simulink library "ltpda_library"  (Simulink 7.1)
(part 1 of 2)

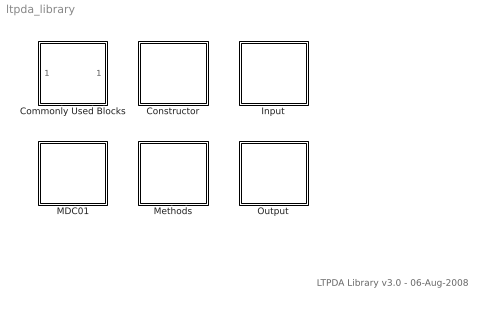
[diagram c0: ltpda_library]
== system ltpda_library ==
  note: LTPDA Library v3.0 - 06-Aug-2008
  Commonly Used Blocks : Subsystem
  Constructor : Subsystem  Tag=subsystem  AncestorBlock=libraryBase/SubSystName
  Input : Subsystem
  MDC01 : Subsystem  Tag=subsystem  AncestorBlock=libraryBase/SubSystName
  Methods : Subsystem  Tag=subsystem  AncestorBlock=libraryBase/SubSystName
  Output : Subsystem

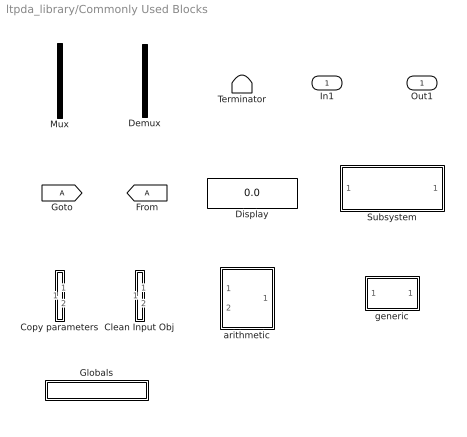
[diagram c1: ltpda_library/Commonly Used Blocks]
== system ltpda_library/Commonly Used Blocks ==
  In1 : Inport  OutDataType=sfix(16)  OutScaling=2^0
  Clean Input Obj : Subsystem
  Copy parameters : Subsystem
  Demux : Demux  Tag=demux  Outputs=2
  Display : Display
  Globals : Subsystem  Tag=globals
  Mux : Mux  Tag=mux  Inputs=2
  Subsystem : Subsystem
  Terminator : Terminator
  arithmetic : Subsystem  Tag=arithmetic
  generic : Subsystem  Tag=function
  Out1 : Outport  OutDataType=sfix(16)  OutScaling=2^0

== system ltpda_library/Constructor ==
  ltpda_getAOsInTimeSpan : Subsystem  Tag=function  AncestorBlock=libraryBase/function

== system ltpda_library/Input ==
  Object from list : Subsystem  Tag=input

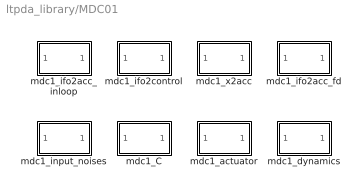
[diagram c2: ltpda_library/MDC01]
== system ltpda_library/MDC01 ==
  mdc1_C : Subsystem  Tag=function  AncestorBlock=libraryBase/function
  mdc1_actuator : Subsystem  Tag=function  AncestorBlock=libraryBase/function
  mdc1_dynamics : Subsystem  Tag=function  AncestorBlock=libraryBase/function
  mdc1_ifo2acc_fd : Subsystem  Tag=function  AncestorBlock=libraryBase/function
  mdc1_ifo2acc_inloop : Subsystem  Tag=function  AncestorBlock=libraryBase/function
  mdc1_ifo2control : Subsystem  Tag=function  AncestorBlock=libraryBase/function
  mdc1_input_noises : Subsystem  Tag=function  AncestorBlock=libraryBase/function
  mdc1_x2acc : Subsystem  Tag=function  AncestorBlock=libraryBase/function

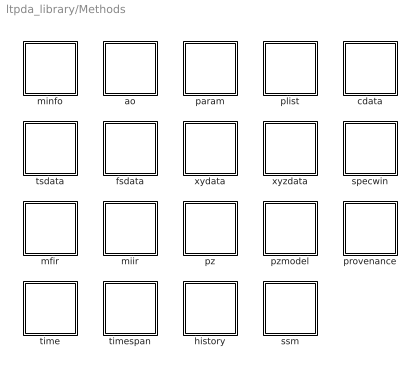
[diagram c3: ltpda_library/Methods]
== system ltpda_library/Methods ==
  ao : Subsystem  Tag=subsystem  AncestorBlock=libraryBase/SubSystName
  cdata : Subsystem  Tag=subsystem  AncestorBlock=libraryBase/SubSystName
  fsdata : Subsystem  Tag=subsystem  AncestorBlock=libraryBase/SubSystName
  history : Subsystem  Tag=subsystem  AncestorBlock=libraryBase/SubSystName
  mfir : Subsystem  Tag=subsystem  AncestorBlock=libraryBase/SubSystName
  miir : Subsystem  Tag=subsystem  AncestorBlock=libraryBase/SubSystName
  minfo : Subsystem  Tag=subsystem  AncestorBlock=libraryBase/SubSystName
  param : Subsystem  Tag=subsystem  AncestorBlock=libraryBase/SubSystName
  plist : Subsystem  Tag=subsystem  AncestorBlock=libraryBase/SubSystName
  provenance : Subsystem  Tag=subsystem  AncestorBlock=libraryBase/SubSystName
  pz : Subsystem  Tag=subsystem  AncestorBlock=libraryBase/SubSystName
  pzmodel : Subsystem  Tag=subsystem  AncestorBlock=libraryBase/SubSystName
  specwin : Subsystem  Tag=subsystem  AncestorBlock=libraryBase/SubSystName
  ssm : Subsystem  Tag=subsystem  AncestorBlock=libraryBase/SubSystName
  time : Subsystem  Tag=subsystem  AncestorBlock=libraryBase/SubSystName
  timespan : Subsystem  Tag=subsystem  AncestorBlock=libraryBase/SubSystName
  tsdata : Subsystem  Tag=subsystem  AncestorBlock=libraryBase/SubSystName
  xydata : Subsystem  Tag=subsystem  AncestorBlock=libraryBase/SubSystName
  xyzdata : Subsystem  Tag=subsystem  AncestorBlock=libraryBase/SubSystName

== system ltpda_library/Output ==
  Send to output : Subsystem
  iplot : Subsystem  Tag=method ao
  plot : Subsystem  Tag=method ao
  save : Subsystem  Tag=method ao

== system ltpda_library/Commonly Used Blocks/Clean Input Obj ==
  In1 : Inport  OutDataType=sfix(16)  OutScaling=2^0
  In2 : Inport  Port=2  OutDataType=sfix(16)  OutScaling=2^0
  cleaninput : M-S-Function  FunctionName=g_cleaninput
  Out1 : Outport  OutDataType=sfix(16)  OutScaling=2^0
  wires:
  In2/1 -> cleaninput/2
  In1/1 -> cleaninput/1
  cleaninput/1 -> Out1/1

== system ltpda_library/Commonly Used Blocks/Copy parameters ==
  In1 : Inport  OutDataType=sfix(16)  OutScaling=2^0
  In2 : Inport  Port=2  OutDataType=sfix(16)  OutScaling=2^0
  copyparam : M-S-Function  FunctionName=g_copyparams
  Out1 : Outport  OutDataType=sfix(16)  OutScaling=2^0
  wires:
  copyparam/1 -> Out1/1
  In1/1 -> copyparam/1
  In2/1 -> copyparam/2

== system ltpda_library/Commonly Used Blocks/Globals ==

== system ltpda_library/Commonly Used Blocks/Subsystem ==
  In1 : Inport  OutDataType=sfix(16)  OutScaling=2^0
  Out1 : Outport  OutDataType=sfix(16)  OutScaling=2^0

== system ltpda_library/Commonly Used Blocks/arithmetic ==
  alpha : Inport  Tag=1  OutDataType=sfix(16)  OutScaling=2^0
  beta : Inport  Tag=2  Port=2  OutDataType=sfix(16)  OutScaling=2^0
  Mux : Mux  Tag=mux  Inputs=2
  arithmetic_func : M-S-Function  Tag=arithmetic  FunctionName=ltpdasim
  Out1 : Outport  OutDataType=sfix(16)  OutScaling=2^0
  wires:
  arithmetic_func/1 -> Out1/1
  Mux/1 -> arithmetic_func/1
  alpha/1 -> Mux/1
  beta/1 -> Mux/2

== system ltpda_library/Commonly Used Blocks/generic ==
  In1 : Inport  OutDataType=sfix(16)  OutScaling=2^0
  generic : M-S-Function  Tag=generic  FunctionName=ltpdasim
  Out1 : Outport  OutDataType=sfix(16)  OutScaling=2^0
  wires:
  generic/1 -> Out1/1
  In1/1 -> generic/1

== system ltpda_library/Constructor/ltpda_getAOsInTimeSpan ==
  In1 : Inport  OutDataType=sfix(16)  OutScaling=2^0
  ltpda_getAOsInTimeSpan : M-S-Function  Tag=ltpda_getAOsInTimeSpan  FunctionName=ltpdasim
  Out1 : Outport  OutDataType=sfix(16)  OutScaling=2^0
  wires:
  In1/1 -> ltpda_getAOsInTimeSpan/1
  ltpda_getAOsInTimeSpan/1 -> Out1/1

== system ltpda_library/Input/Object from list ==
  Input : Constant  Value=0  OutDataType=sfix(16)  OutScaling=2^0
  Input AO : Outport  OutDataType=sfix(16)  OutScaling=2^0
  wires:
  Input/1 -> Input AO/1

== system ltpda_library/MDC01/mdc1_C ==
  In1 : Inport  OutDataType=sfix(16)  OutScaling=2^0
  ltpda_mdc1_C : M-S-Function  Tag=ltpda_mdc1_C  FunctionName=ltpdasim
  Out1 : Outport  OutDataType=sfix(16)  OutScaling=2^0
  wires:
  In1/1 -> ltpda_mdc1_C/1
  ltpda_mdc1_C/1 -> Out1/1

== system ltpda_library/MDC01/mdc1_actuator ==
  In1 : Inport  OutDataType=sfix(16)  OutScaling=2^0
  ltpda_mdc1_actuator : M-S-Function  Tag=ltpda_mdc1_actuator  FunctionName=ltpdasim
  Out1 : Outport  OutDataType=sfix(16)  OutScaling=2^0
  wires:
  In1/1 -> ltpda_mdc1_actuator/1
  ltpda_mdc1_actuator/1 -> Out1/1

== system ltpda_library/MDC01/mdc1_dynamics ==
  In1 : Inport  OutDataType=sfix(16)  OutScaling=2^0
  ltpda_mdc1_dynamics : M-S-Function  Tag=ltpda_mdc1_dynamics  FunctionName=ltpdasim
  Out1 : Outport  OutDataType=sfix(16)  OutScaling=2^0
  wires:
  In1/1 -> ltpda_mdc1_dynamics/1
  ltpda_mdc1_dynamics/1 -> Out1/1

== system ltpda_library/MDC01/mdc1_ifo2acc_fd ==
  In1 : Inport  OutDataType=sfix(16)  OutScaling=2^0
  ltpda_mdc1_ifo2acc_fd : M-S-Function  Tag=ltpda_mdc1_ifo2acc_fd  FunctionName=ltpdasim
  Out1 : Outport  OutDataType=sfix(16)  OutScaling=2^0
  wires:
  In1/1 -> ltpda_mdc1_ifo2acc_fd/1
  ltpda_mdc1_ifo2acc_fd/1 -> Out1/1

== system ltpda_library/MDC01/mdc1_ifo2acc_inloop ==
  In1 : Inport  OutDataType=sfix(16)  OutScaling=2^0
  ltpda_mdc1_ifo2acc_inloop : M-S-Function  Tag=ltpda_mdc1_ifo2acc_inloop  FunctionName=ltpdasim
  Out1 : Outport  OutDataType=sfix(16)  OutScaling=2^0
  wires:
  In1/1 -> ltpda_mdc1_ifo2acc_inloop/1
  ltpda_mdc1_ifo2acc_inloop/1 -> Out1/1

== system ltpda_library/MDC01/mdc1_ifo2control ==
  In1 : Inport  OutDataType=sfix(16)  OutScaling=2^0
  ltpda_mdc1_ifo2control : M-S-Function  Tag=ltpda_mdc1_ifo2control  FunctionName=ltpdasim
  Out1 : Outport  OutDataType=sfix(16)  OutScaling=2^0
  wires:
  In1/1 -> ltpda_mdc1_ifo2control/1
  ltpda_mdc1_ifo2control/1 -> Out1/1

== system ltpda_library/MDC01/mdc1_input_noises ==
  In1 : Inport  OutDataType=sfix(16)  OutScaling=2^0
  ltpda_mdc1_input_noises : M-S-Function  Tag=ltpda_mdc1_input_noises  FunctionName=ltpdasim
  Out1 : Outport  OutDataType=sfix(16)  OutScaling=2^0
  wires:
  In1/1 -> ltpda_mdc1_input_noises/1
  ltpda_mdc1_input_noises/1 -> Out1/1

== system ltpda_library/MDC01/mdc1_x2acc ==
  In1 : Inport  OutDataType=sfix(16)  OutScaling=2^0
  ltpda_mdc1_x2acc : M-S-Function  Tag=ltpda_mdc1_x2acc  FunctionName=ltpdasim
  Out1 : Outport  OutDataType=sfix(16)  OutScaling=2^0
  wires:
  In1/1 -> ltpda_mdc1_x2acc/1
  ltpda_mdc1_x2acc/1 -> Out1/1

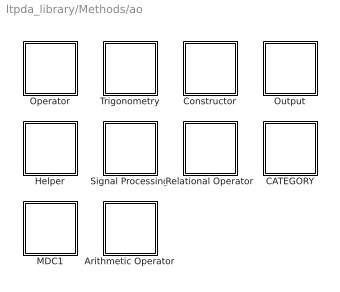
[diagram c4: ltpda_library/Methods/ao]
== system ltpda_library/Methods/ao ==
  Arithmetic Operator : Subsystem  Tag=subsystem  AncestorBlock=libraryBase/SubSystName
  CATEGORY : Subsystem  Tag=subsystem  AncestorBlock=libraryBase/SubSystName
  Constructor : Subsystem  Tag=subsystem  AncestorBlock=libraryBase/SubSystName
  Helper : Subsystem  Tag=subsystem  AncestorBlock=libraryBase/SubSystName
  MDC1 : Subsystem  Tag=subsystem  AncestorBlock=libraryBase/SubSystName
  Operator : Subsystem  Tag=subsystem  AncestorBlock=libraryBase/SubSystName
  Output : Subsystem  Tag=subsystem  AncestorBlock=libraryBase/SubSystName
  Relational Operator : Subsystem  Tag=subsystem  AncestorBlock=libraryBase/SubSystName
  Signal Processing : Subsystem  Tag=subsystem  AncestorBlock=libraryBase/SubSystName
  Trigonometry : Subsystem  Tag=subsystem  AncestorBlock=libraryBase/SubSystName

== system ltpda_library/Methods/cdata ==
  Constructor : Subsystem  Tag=subsystem  AncestorBlock=libraryBase/SubSystName
  Output : Subsystem  Tag=subsystem  AncestorBlock=libraryBase/SubSystName

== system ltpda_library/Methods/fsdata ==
  Constructor : Subsystem  Tag=subsystem  AncestorBlock=libraryBase/SubSystName
  Output : Subsystem  Tag=subsystem  AncestorBlock=libraryBase/SubSystName

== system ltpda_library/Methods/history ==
  Constructor : Subsystem  Tag=subsystem  AncestorBlock=libraryBase/SubSystName
  Output : Subsystem  Tag=subsystem  AncestorBlock=libraryBase/SubSystName

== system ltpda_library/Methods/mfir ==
  Constructor : Subsystem  Tag=subsystem  AncestorBlock=libraryBase/SubSystName
  Helper : Subsystem  Tag=subsystem  AncestorBlock=libraryBase/SubSystName
  Output : Subsystem  Tag=subsystem  AncestorBlock=libraryBase/SubSystName
  Signal Processing : Subsystem  Tag=subsystem  AncestorBlock=libraryBase/SubSystName

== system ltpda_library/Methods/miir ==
  Constructor : Subsystem  Tag=subsystem  AncestorBlock=libraryBase/SubSystName
  Helper : Subsystem  Tag=subsystem  AncestorBlock=libraryBase/SubSystName
  Output : Subsystem  Tag=subsystem  AncestorBlock=libraryBase/SubSystName
  Signal Processing : Subsystem  Tag=subsystem  AncestorBlock=libraryBase/SubSystName

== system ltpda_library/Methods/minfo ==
  Constructor : Subsystem  Tag=subsystem  AncestorBlock=libraryBase/SubSystName
  Output : Subsystem  Tag=subsystem  AncestorBlock=libraryBase/SubSystName

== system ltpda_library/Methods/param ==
  Constructor : Subsystem  Tag=subsystem  AncestorBlock=libraryBase/SubSystName
  Helper : Subsystem  Tag=subsystem  AncestorBlock=libraryBase/SubSystName
  Output : Subsystem  Tag=subsystem  AncestorBlock=libraryBase/SubSystName

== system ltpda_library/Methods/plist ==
  Constructor : Subsystem  Tag=subsystem  AncestorBlock=libraryBase/SubSystName
  Helper : Subsystem  Tag=subsystem  AncestorBlock=libraryBase/SubSystName
  Output : Subsystem  Tag=subsystem  AncestorBlock=libraryBase/SubSystName
  Signal Processing : Subsystem  Tag=subsystem  AncestorBlock=libraryBase/SubSystName

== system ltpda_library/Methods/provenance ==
  Constructor : Subsystem  Tag=subsystem  AncestorBlock=libraryBase/SubSystName
  Output : Subsystem  Tag=subsystem  AncestorBlock=libraryBase/SubSystName

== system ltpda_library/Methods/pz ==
  Constructor : Subsystem  Tag=subsystem  AncestorBlock=libraryBase/SubSystName
  Output : Subsystem  Tag=subsystem  AncestorBlock=libraryBase/SubSystName
  Signal Processing : Subsystem  Tag=subsystem  AncestorBlock=libraryBase/SubSystName

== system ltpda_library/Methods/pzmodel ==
  Constructor : Subsystem  Tag=subsystem  AncestorBlock=libraryBase/SubSystName
  Helper : Subsystem  Tag=subsystem  AncestorBlock=libraryBase/SubSystName
  Operator : Subsystem  Tag=subsystem  AncestorBlock=libraryBase/SubSystName
  Output : Subsystem  Tag=subsystem  AncestorBlock=libraryBase/SubSystName
  Signal Processing : Subsystem  Tag=subsystem  AncestorBlock=libraryBase/SubSystName

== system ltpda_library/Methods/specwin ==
  Constructor : Subsystem  Tag=subsystem  AncestorBlock=libraryBase/SubSystName
  Output : Subsystem  Tag=subsystem  AncestorBlock=libraryBase/SubSystName

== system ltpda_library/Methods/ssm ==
  Constructor : Subsystem  Tag=subsystem  AncestorBlock=libraryBase/SubSystName

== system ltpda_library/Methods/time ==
  Arithmetic Operator : Subsystem  Tag=subsystem  AncestorBlock=libraryBase/SubSystName
  Constructor : Subsystem  Tag=subsystem  AncestorBlock=libraryBase/SubSystName
  Helper : Subsystem  Tag=subsystem  AncestorBlock=libraryBase/SubSystName
  Output : Subsystem  Tag=subsystem  AncestorBlock=libraryBase/SubSystName

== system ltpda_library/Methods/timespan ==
  Constructor : Subsystem  Tag=subsystem  AncestorBlock=libraryBase/SubSystName
  Helper : Subsystem  Tag=subsystem  AncestorBlock=libraryBase/SubSystName
  Output : Subsystem  Tag=subsystem  AncestorBlock=libraryBase/SubSystName

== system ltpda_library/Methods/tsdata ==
  Constructor : Subsystem  Tag=subsystem  AncestorBlock=libraryBase/SubSystName
  Output : Subsystem  Tag=subsystem  AncestorBlock=libraryBase/SubSystName

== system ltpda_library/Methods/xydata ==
  Constructor : Subsystem  Tag=subsystem  AncestorBlock=libraryBase/SubSystName
  Output : Subsystem  Tag=subsystem  AncestorBlock=libraryBase/SubSystName

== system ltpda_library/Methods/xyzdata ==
  Constructor : Subsystem  Tag=subsystem  AncestorBlock=libraryBase/SubSystName
  Output : Subsystem  Tag=subsystem  AncestorBlock=libraryBase/SubSystName

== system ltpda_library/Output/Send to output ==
  In1 : Inport  OutDataType=sfix(16)  OutScaling=2^0
  save result : M-S-Function  FunctionName=g_saveresult
  Out1 : Outport  OutDataType=sfix(16)  OutScaling=2^0
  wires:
  In1/1 -> save result/1
  save result/1 -> Out1/1

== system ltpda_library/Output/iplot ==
  In1 : Inport  OutDataType=sfix(16)  OutScaling=2^0
  Terminator : Terminator
  iplot : M-S-Function  Tag=iplot  FunctionName=ltpdasim
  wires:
  In1/1 -> iplot/1
  iplot/1 -> Terminator/1

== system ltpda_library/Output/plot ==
  In1 : Inport  OutDataType=sfix(16)  OutScaling=2^0
  Terminator : Terminator
  plot : M-S-Function  Tag=plot  FunctionName=ltpdasim
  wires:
  In1/1 -> plot/1
  plot/1 -> Terminator/1

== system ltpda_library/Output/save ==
  In1 : Inport  OutDataType=sfix(16)  OutScaling=2^0
  Terminator : Terminator
  save : M-S-Function  Tag=save  FunctionName=ltpdasim
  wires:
  In1/1 -> save/1
  save/1 -> Terminator/1

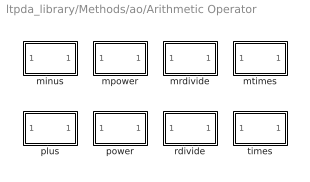
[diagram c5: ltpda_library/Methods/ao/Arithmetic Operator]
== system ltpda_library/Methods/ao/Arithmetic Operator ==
  minus : Subsystem  Tag=method ao  AncestorBlock=libraryBase/function
  mpower : Subsystem  Tag=method ao  AncestorBlock=libraryBase/function
  mrdivide : Subsystem  Tag=method ao  AncestorBlock=libraryBase/function
  mtimes : Subsystem  Tag=method ao  AncestorBlock=libraryBase/function
  plus : Subsystem  Tag=method ao  AncestorBlock=libraryBase/function
  power : Subsystem  Tag=method ao  AncestorBlock=libraryBase/function
  rdivide : Subsystem  Tag=method ao  AncestorBlock=libraryBase/function
  times : Subsystem  Tag=method ao  AncestorBlock=libraryBase/function

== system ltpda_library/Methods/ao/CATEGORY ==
  lincom : Subsystem  Tag=method ao  AncestorBlock=libraryBase/function
  timedomainfit : Subsystem  Tag=method ao  AncestorBlock=libraryBase/function

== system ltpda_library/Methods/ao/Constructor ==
  ao : Subsystem  Tag=method ao  AncestorBlock=libraryBase/constructor

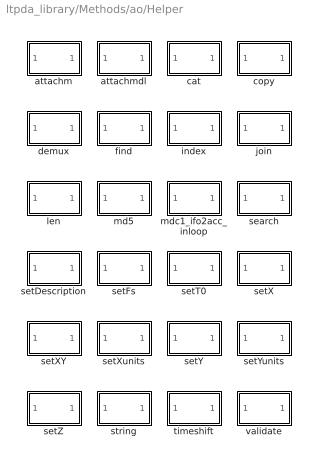
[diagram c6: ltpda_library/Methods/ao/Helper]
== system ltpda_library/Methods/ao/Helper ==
  attachm : Subsystem  Tag=method ao  AncestorBlock=libraryBase/function
  attachmdl : Subsystem  Tag=method ao  AncestorBlock=libraryBase/function
  cat : Subsystem  Tag=method ao  AncestorBlock=libraryBase/function
  copy : Subsystem  Tag=method ao  AncestorBlock=libraryBase/function
  demux : Subsystem  Tag=method ao  AncestorBlock=libraryBase/function
  find : Subsystem  Tag=method ao  AncestorBlock=libraryBase/function
  index : Subsystem  Tag=method ao  AncestorBlock=libraryBase/function
  join : Subsystem  Tag=method ao  AncestorBlock=libraryBase/function
  len : Subsystem  Tag=method ao  AncestorBlock=libraryBase/function
  md5 : Subsystem  Tag=method ao  AncestorBlock=libraryBase/function
  mdc1_ifo2acc_inloop : Subsystem  Tag=method ao  AncestorBlock=libraryBase/function
  search : Subsystem  Tag=method ao  AncestorBlock=libraryBase/function
  setDescription : Subsystem  Tag=method ao  AncestorBlock=libraryBase/function
  setFs : Subsystem  Tag=method ao  AncestorBlock=libraryBase/function
  setT0 : Subsystem  Tag=method ao  AncestorBlock=libraryBase/function
  setX : Subsystem  Tag=method ao  AncestorBlock=libraryBase/function
  setXY : Subsystem  Tag=method ao  AncestorBlock=libraryBase/function
  setXunits : Subsystem  Tag=method ao  AncestorBlock=libraryBase/function
  setY : Subsystem  Tag=method ao  AncestorBlock=libraryBase/function
  setYunits : Subsystem  Tag=method ao  AncestorBlock=libraryBase/function
  setZ : Subsystem  Tag=method ao  AncestorBlock=libraryBase/function
  string : Subsystem  Tag=method ao  AncestorBlock=libraryBase/function
  timeshift : Subsystem  Tag=method ao  AncestorBlock=libraryBase/function
  validate : Subsystem  Tag=method ao  AncestorBlock=libraryBase/function

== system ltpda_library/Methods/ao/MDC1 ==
  mdc1_ifo2control : Subsystem  Tag=method ao  AncestorBlock=libraryBase/function
  mdc1_x2acc : Subsystem  Tag=method ao  AncestorBlock=libraryBase/function

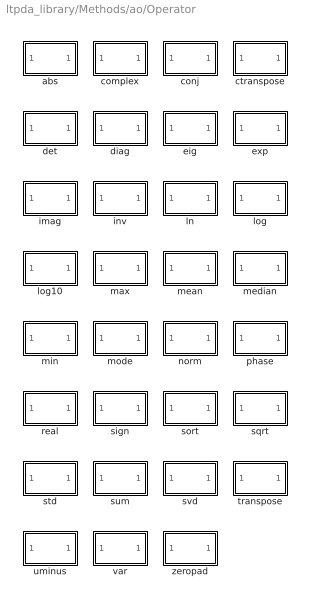
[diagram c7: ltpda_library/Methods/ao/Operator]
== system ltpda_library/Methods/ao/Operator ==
  abs : Subsystem  Tag=method ao  AncestorBlock=libraryBase/function
  complex : Subsystem  Tag=method ao  AncestorBlock=libraryBase/function
  conj : Subsystem  Tag=method ao  AncestorBlock=libraryBase/function
  ctranspose : Subsystem  Tag=method ao  AncestorBlock=libraryBase/function
  det : Subsystem  Tag=method ao  AncestorBlock=libraryBase/function
  diag : Subsystem  Tag=method ao  AncestorBlock=libraryBase/function
  eig : Subsystem  Tag=method ao  AncestorBlock=libraryBase/function
  exp : Subsystem  Tag=method ao  AncestorBlock=libraryBase/function
  imag : Subsystem  Tag=method ao  AncestorBlock=libraryBase/function
  inv : Subsystem  Tag=method ao  AncestorBlock=libraryBase/function
  ln : Subsystem  Tag=method ao  AncestorBlock=libraryBase/function
  log : Subsystem  Tag=method ao  AncestorBlock=libraryBase/function
  log10 : Subsystem  Tag=method ao  AncestorBlock=libraryBase/function
  max : Subsystem  Tag=method ao  AncestorBlock=libraryBase/function
  mean : Subsystem  Tag=method ao  AncestorBlock=libraryBase/function
  median : Subsystem  Tag=method ao  AncestorBlock=libraryBase/function
  min : Subsystem  Tag=method ao  AncestorBlock=libraryBase/function
  mode : Subsystem  Tag=method ao  AncestorBlock=libraryBase/function
  norm : Subsystem  Tag=method ao  AncestorBlock=libraryBase/function
  phase : Subsystem  Tag=method ao  AncestorBlock=libraryBase/function
  real : Subsystem  Tag=method ao  AncestorBlock=libraryBase/function
  sign : Subsystem  Tag=method ao  AncestorBlock=libraryBase/function
  sort : Subsystem  Tag=method ao  AncestorBlock=libraryBase/function
  sqrt : Subsystem  Tag=method ao  AncestorBlock=libraryBase/function
  std : Subsystem  Tag=method ao  AncestorBlock=libraryBase/function
  sum : Subsystem  Tag=method ao  AncestorBlock=libraryBase/function
  svd : Subsystem  Tag=method ao  AncestorBlock=libraryBase/function
  transpose : Subsystem  Tag=method ao  AncestorBlock=libraryBase/function
  uminus : Subsystem  Tag=method ao  AncestorBlock=libraryBase/function
  var : Subsystem  Tag=method ao  AncestorBlock=libraryBase/function
  zeropad : Subsystem  Tag=method ao  AncestorBlock=libraryBase/function

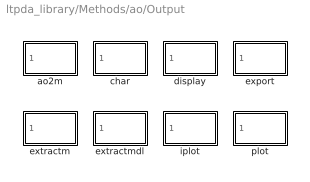
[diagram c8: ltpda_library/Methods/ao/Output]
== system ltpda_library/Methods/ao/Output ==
  ao2m : Subsystem  Tag=method ao  AncestorBlock=libraryBase/output
  char : Subsystem  Tag=method ao  AncestorBlock=libraryBase/output
  display : Subsystem  Tag=method ao  AncestorBlock=libraryBase/output
  export : Subsystem  Tag=method ao  AncestorBlock=libraryBase/output
  extractm : Subsystem  Tag=method ao  AncestorBlock=libraryBase/output
  extractmdl : Subsystem  Tag=method ao  AncestorBlock=libraryBase/output
  iplot : Subsystem  Tag=method ao  AncestorBlock=libraryBase/output
  plot : Subsystem  Tag=method ao  AncestorBlock=libraryBase/output

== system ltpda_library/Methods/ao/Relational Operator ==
  ge : Subsystem  Tag=method ao  AncestorBlock=libraryBase/function
  gt : Subsystem  Tag=method ao  AncestorBlock=libraryBase/function
  le : Subsystem  Tag=method ao  AncestorBlock=libraryBase/function
  lt : Subsystem  Tag=method ao  AncestorBlock=libraryBase/function

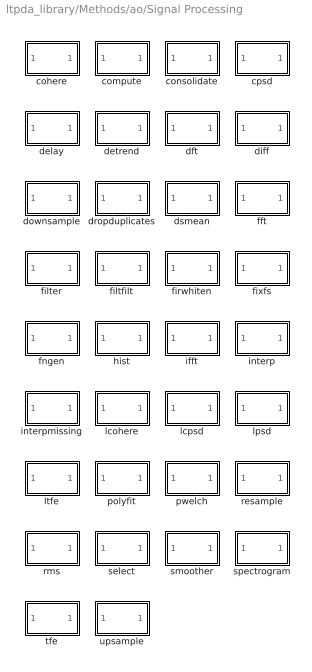
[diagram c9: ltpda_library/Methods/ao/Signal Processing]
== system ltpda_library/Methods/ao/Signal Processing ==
  cohere : Subsystem  Tag=method ao  AncestorBlock=libraryBase/function
  compute : Subsystem  Tag=method ao  AncestorBlock=libraryBase/function
  consolidate : Subsystem  Tag=method ao  AncestorBlock=libraryBase/function
  cpsd : Subsystem  Tag=method ao  AncestorBlock=libraryBase/function
  delay : Subsystem  Tag=method ao  AncestorBlock=libraryBase/function
  detrend : Subsystem  Tag=method ao  AncestorBlock=libraryBase/function
  dft : Subsystem  Tag=method ao  AncestorBlock=libraryBase/function
  diff : Subsystem  Tag=method ao  AncestorBlock=libraryBase/function
  downsample : Subsystem  Tag=method ao  AncestorBlock=libraryBase/function
  dropduplicates : Subsystem  Tag=method ao  AncestorBlock=libraryBase/function
  dsmean : Subsystem  Tag=method ao  AncestorBlock=libraryBase/function
  fft : Subsystem  Tag=method ao  AncestorBlock=libraryBase/function
  filter : Subsystem  Tag=method ao  AncestorBlock=libraryBase/function
  filtfilt : Subsystem  Tag=method ao  AncestorBlock=libraryBase/function
  firwhiten : Subsystem  Tag=method ao  AncestorBlock=libraryBase/function
  fixfs : Subsystem  Tag=method ao  AncestorBlock=libraryBase/function
  fngen : Subsystem  Tag=method ao  AncestorBlock=libraryBase/function
  hist : Subsystem  Tag=method ao  AncestorBlock=libraryBase/function
  ifft : Subsystem  Tag=method ao  AncestorBlock=libraryBase/function
  interp : Subsystem  Tag=method ao  AncestorBlock=libraryBase/function
  interpmissing : Subsystem  Tag=method ao  AncestorBlock=libraryBase/function
  lcohere : Subsystem  Tag=method ao  AncestorBlock=libraryBase/function
  lcpsd : Subsystem  Tag=method ao  AncestorBlock=libraryBase/function
  lpsd : Subsystem  Tag=method ao  AncestorBlock=libraryBase/function
  ltfe : Subsystem  Tag=method ao  AncestorBlock=libraryBase/function
  polyfit : Subsystem  Tag=method ao  AncestorBlock=libraryBase/function
  pwelch : Subsystem  Tag=method ao  AncestorBlock=libraryBase/function
  resample : Subsystem  Tag=method ao  AncestorBlock=libraryBase/function
  rms : Subsystem  Tag=method ao  AncestorBlock=libraryBase/function
  select : Subsystem  Tag=method ao  AncestorBlock=libraryBase/function
  smoother : Subsystem  Tag=method ao  AncestorBlock=libraryBase/function
  spectrogram : Subsystem  Tag=method ao  AncestorBlock=libraryBase/function
  tfe : Subsystem  Tag=method ao  AncestorBlock=libraryBase/function
  upsample : Subsystem  Tag=method ao  AncestorBlock=libraryBase/function

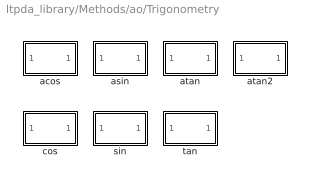
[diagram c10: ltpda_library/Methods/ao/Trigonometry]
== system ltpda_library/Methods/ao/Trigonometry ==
  acos : Subsystem  Tag=method ao  AncestorBlock=libraryBase/function
  asin : Subsystem  Tag=method ao  AncestorBlock=libraryBase/function
  atan : Subsystem  Tag=method ao  AncestorBlock=libraryBase/function
  atan2 : Subsystem  Tag=method ao  AncestorBlock=libraryBase/function
  cos : Subsystem  Tag=method ao  AncestorBlock=libraryBase/function
  sin : Subsystem  Tag=method ao  AncestorBlock=libraryBase/function
  tan : Subsystem  Tag=method ao  AncestorBlock=libraryBase/function

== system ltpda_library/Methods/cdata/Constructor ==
  cdata : Subsystem  Tag=method cdata  AncestorBlock=libraryBase/constructor

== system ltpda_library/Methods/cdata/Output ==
  display : Subsystem  Tag=method cdata  AncestorBlock=libraryBase/output

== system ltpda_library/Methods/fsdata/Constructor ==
  fsdata : Subsystem  Tag=method fsdata  AncestorBlock=libraryBase/constructor

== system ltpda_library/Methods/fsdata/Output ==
  display : Subsystem  Tag=method fsdata  AncestorBlock=libraryBase/output

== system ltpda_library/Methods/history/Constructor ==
  history : Subsystem  Tag=method history  AncestorBlock=libraryBase/constructor

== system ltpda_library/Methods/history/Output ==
  char : Subsystem  Tag=method history  AncestorBlock=libraryBase/output
  display : Subsystem  Tag=method history  AncestorBlock=libraryBase/output
  hist2dot : Subsystem  Tag=method history  AncestorBlock=libraryBase/output
  hist2m : Subsystem  Tag=method history  AncestorBlock=libraryBase/output
  plot : Subsystem  Tag=method history  AncestorBlock=libraryBase/output
  string : Subsystem  Tag=method history  AncestorBlock=libraryBase/output

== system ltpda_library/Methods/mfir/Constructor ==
  mfir : Subsystem  Tag=method mfir  AncestorBlock=libraryBase/constructor

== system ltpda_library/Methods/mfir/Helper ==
  redesign : Subsystem  Tag=method mfir  AncestorBlock=libraryBase/function

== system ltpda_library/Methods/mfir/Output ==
  char : Subsystem  Tag=method mfir  AncestorBlock=libraryBase/output
  display : Subsystem  Tag=method mfir  AncestorBlock=libraryBase/output
  string : Subsystem  Tag=method mfir  AncestorBlock=libraryBase/output

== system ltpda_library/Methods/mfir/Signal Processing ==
  resp : Subsystem  Tag=method mfir  AncestorBlock=libraryBase/function

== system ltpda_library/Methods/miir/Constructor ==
  miir : Subsystem  Tag=method miir  AncestorBlock=libraryBase/constructor

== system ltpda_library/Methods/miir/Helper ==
  redesign : Subsystem  Tag=method miir  AncestorBlock=libraryBase/function

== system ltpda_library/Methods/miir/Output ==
  char : Subsystem  Tag=method miir  AncestorBlock=libraryBase/output
  display : Subsystem  Tag=method miir  AncestorBlock=libraryBase/output
  string : Subsystem  Tag=method miir  AncestorBlock=libraryBase/output

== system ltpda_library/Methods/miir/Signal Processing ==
  resp : Subsystem  Tag=method miir  AncestorBlock=libraryBase/function

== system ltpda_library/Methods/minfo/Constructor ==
  minfo : Subsystem  Tag=method minfo  AncestorBlock=libraryBase/constructor

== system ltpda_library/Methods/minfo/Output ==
  char : Subsystem  Tag=method minfo  AncestorBlock=libraryBase/output
  display : Subsystem  Tag=method minfo  AncestorBlock=libraryBase/output

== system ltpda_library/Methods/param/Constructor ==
  param : Subsystem  Tag=method param  AncestorBlock=libraryBase/constructor

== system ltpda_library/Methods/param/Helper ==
  mux : Subsystem  Tag=method param  AncestorBlock=libraryBase/function

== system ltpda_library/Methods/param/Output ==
  char : Subsystem  Tag=method param  AncestorBlock=libraryBase/output
  display : Subsystem  Tag=method param  AncestorBlock=libraryBase/output
  display2 : Subsystem  Tag=method param  AncestorBlock=libraryBase/output
  string : Subsystem  Tag=method param  AncestorBlock=libraryBase/output

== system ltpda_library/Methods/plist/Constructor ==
  plist : Subsystem  Tag=method plist  AncestorBlock=libraryBase/constructor

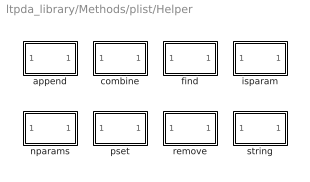
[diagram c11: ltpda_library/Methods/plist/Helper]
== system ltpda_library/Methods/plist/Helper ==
  append : Subsystem  Tag=method plist  AncestorBlock=libraryBase/function
  combine : Subsystem  Tag=method plist  AncestorBlock=libraryBase/function
  find : Subsystem  Tag=method plist  AncestorBlock=libraryBase/function
  isparam : Subsystem  Tag=method plist  AncestorBlock=libraryBase/function
  nparams : Subsystem  Tag=method plist  AncestorBlock=libraryBase/function
  pset : Subsystem  Tag=method plist  AncestorBlock=libraryBase/function
  remove : Subsystem  Tag=method plist  AncestorBlock=libraryBase/function
  string : Subsystem  Tag=method plist  AncestorBlock=libraryBase/function

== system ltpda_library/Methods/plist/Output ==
  char : Subsystem  Tag=method plist  AncestorBlock=libraryBase/output
  display : Subsystem  Tag=method plist  AncestorBlock=libraryBase/output

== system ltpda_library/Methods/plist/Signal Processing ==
  pzmresp : Subsystem  Tag=method plist  AncestorBlock=libraryBase/function
  resp : Subsystem  Tag=method plist  AncestorBlock=libraryBase/function

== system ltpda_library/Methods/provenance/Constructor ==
  provenance : Subsystem  Tag=method provenance  AncestorBlock=libraryBase/constructor

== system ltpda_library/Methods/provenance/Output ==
  char : Subsystem  Tag=method provenance  AncestorBlock=libraryBase/output
  display : Subsystem  Tag=method provenance  AncestorBlock=libraryBase/output
  string : Subsystem  Tag=method provenance  AncestorBlock=libraryBase/output

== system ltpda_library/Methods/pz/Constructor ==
  pz : Subsystem  Tag=method pz  AncestorBlock=libraryBase/constructor

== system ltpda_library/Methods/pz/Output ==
  char : Subsystem  Tag=method pz  AncestorBlock=libraryBase/output
  display : Subsystem  Tag=method pz  AncestorBlock=libraryBase/output
  string : Subsystem  Tag=method pz  AncestorBlock=libraryBase/output

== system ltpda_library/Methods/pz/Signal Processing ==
  resp : Subsystem  Tag=method pz  AncestorBlock=libraryBase/function

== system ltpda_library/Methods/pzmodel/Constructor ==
  pzmodel : Subsystem  Tag=method pzmodel  AncestorBlock=libraryBase/constructor

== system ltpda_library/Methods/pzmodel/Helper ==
  string : Subsystem  Tag=method pzmodel  AncestorBlock=libraryBase/function

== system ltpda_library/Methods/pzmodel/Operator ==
  tomfir : Subsystem  Tag=method pzmodel  AncestorBlock=libraryBase/function
  tomiir : Subsystem  Tag=method pzmodel  AncestorBlock=libraryBase/function

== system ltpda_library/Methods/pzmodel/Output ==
  char : Subsystem  Tag=method pzmodel  AncestorBlock=libraryBase/output
  display : Subsystem  Tag=method pzmodel  AncestorBlock=libraryBase/output

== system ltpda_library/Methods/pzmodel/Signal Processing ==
  fngen : Subsystem  Tag=method pzmodel  AncestorBlock=libraryBase/function
  resp : Subsystem  Tag=method pzmodel  AncestorBlock=libraryBase/function

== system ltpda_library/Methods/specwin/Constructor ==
  specwin : Subsystem  Tag=method specwin  AncestorBlock=libraryBase/constructor

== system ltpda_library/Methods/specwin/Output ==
  char : Subsystem  Tag=method specwin  AncestorBlock=libraryBase/output
  display : Subsystem  Tag=method specwin  AncestorBlock=libraryBase/output
  plot : Subsystem  Tag=method specwin  AncestorBlock=libraryBase/output
  string : Subsystem  Tag=method specwin  AncestorBlock=libraryBase/output

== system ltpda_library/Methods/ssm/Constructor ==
  ssm : Subsystem  Tag=method ssm  AncestorBlock=libraryBase/constructor

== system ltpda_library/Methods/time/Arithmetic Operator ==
  minus : Subsystem  Tag=method time  AncestorBlock=libraryBase/function
  plus : Subsystem  Tag=method time  AncestorBlock=libraryBase/function

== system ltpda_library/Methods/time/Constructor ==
  time : Subsystem  Tag=method time  AncestorBlock=libraryBase/constructor

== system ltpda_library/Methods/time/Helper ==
  string : Subsystem  Tag=method time  AncestorBlock=libraryBase/function

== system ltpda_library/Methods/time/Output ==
  char : Subsystem  Tag=method time  AncestorBlock=libraryBase/output
  display : Subsystem  Tag=method time  AncestorBlock=libraryBase/output
  format : Subsystem  Tag=method time  AncestorBlock=libraryBase/output

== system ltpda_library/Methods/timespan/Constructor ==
  timespan : Subsystem  Tag=method timespan  AncestorBlock=libraryBase/constructor

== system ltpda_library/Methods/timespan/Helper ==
  setEndT : Subsystem  Tag=method timespan  AncestorBlock=libraryBase/function
  setStartT : Subsystem  Tag=method timespan  AncestorBlock=libraryBase/function
  setTimeformat : Subsystem  Tag=method timespan  AncestorBlock=libraryBase/function
  setTimezone : Subsystem  Tag=method timespan  AncestorBlock=libraryBase/function

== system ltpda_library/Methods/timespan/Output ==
  char : Subsystem  Tag=method timespan  AncestorBlock=libraryBase/output
  display : Subsystem  Tag=method timespan  AncestorBlock=libraryBase/output
  string : Subsystem  Tag=method timespan  AncestorBlock=libraryBase/output

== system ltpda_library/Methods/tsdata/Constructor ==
  tsdata : Subsystem  Tag=method tsdata  AncestorBlock=libraryBase/constructor

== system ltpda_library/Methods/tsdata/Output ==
  display : Subsystem  Tag=method tsdata  AncestorBlock=libraryBase/output

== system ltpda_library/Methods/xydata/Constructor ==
  xydata : Subsystem  Tag=method xydata  AncestorBlock=libraryBase/constructor

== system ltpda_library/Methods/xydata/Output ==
  display : Subsystem  Tag=method xydata  AncestorBlock=libraryBase/output

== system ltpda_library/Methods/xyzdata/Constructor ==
  xyzdata : Subsystem  Tag=method xyzdata  AncestorBlock=libraryBase/constructor

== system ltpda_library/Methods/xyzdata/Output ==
  char : Subsystem  Tag=method xyzdata  AncestorBlock=libraryBase/output
  display : Subsystem  Tag=method xyzdata  AncestorBlock=libraryBase/output

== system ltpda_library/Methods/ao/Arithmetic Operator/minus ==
  In1 : Inport  OutDataType=sfix(16)  OutScaling=2^0
  minus : M-S-Function  Tag=minus  FunctionName=ltpdasim
  Out1 : Outport  OutDataType=sfix(16)  OutScaling=2^0
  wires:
  In1/1 -> minus/1
  minus/1 -> Out1/1

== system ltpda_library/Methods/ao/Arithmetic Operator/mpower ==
  In1 : Inport  OutDataType=sfix(16)  OutScaling=2^0
  mpower : M-S-Function  Tag=mpower  FunctionName=ltpdasim
  Out1 : Outport  OutDataType=sfix(16)  OutScaling=2^0
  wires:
  In1/1 -> mpower/1
  mpower/1 -> Out1/1

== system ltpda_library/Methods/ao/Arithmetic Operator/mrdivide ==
  In1 : Inport  OutDataType=sfix(16)  OutScaling=2^0
  mrdivide : M-S-Function  Tag=mrdivide  FunctionName=ltpdasim
  Out1 : Outport  OutDataType=sfix(16)  OutScaling=2^0
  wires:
  In1/1 -> mrdivide/1
  mrdivide/1 -> Out1/1

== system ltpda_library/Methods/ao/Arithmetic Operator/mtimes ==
  In1 : Inport  OutDataType=sfix(16)  OutScaling=2^0
  mtimes : M-S-Function  Tag=mtimes  FunctionName=ltpdasim
  Out1 : Outport  OutDataType=sfix(16)  OutScaling=2^0
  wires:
  In1/1 -> mtimes/1
  mtimes/1 -> Out1/1

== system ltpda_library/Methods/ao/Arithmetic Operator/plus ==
  In1 : Inport  OutDataType=sfix(16)  OutScaling=2^0
  plus : M-S-Function  Tag=plus  FunctionName=ltpdasim
  Out1 : Outport  OutDataType=sfix(16)  OutScaling=2^0
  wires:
  In1/1 -> plus/1
  plus/1 -> Out1/1

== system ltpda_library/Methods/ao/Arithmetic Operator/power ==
  In1 : Inport  OutDataType=sfix(16)  OutScaling=2^0
  power : M-S-Function  Tag=power  FunctionName=ltpdasim
  Out1 : Outport  OutDataType=sfix(16)  OutScaling=2^0
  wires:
  In1/1 -> power/1
  power/1 -> Out1/1

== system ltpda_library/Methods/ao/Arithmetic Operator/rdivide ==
  In1 : Inport  OutDataType=sfix(16)  OutScaling=2^0
  rdivide : M-S-Function  Tag=rdivide  FunctionName=ltpdasim
  Out1 : Outport  OutDataType=sfix(16)  OutScaling=2^0
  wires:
  In1/1 -> rdivide/1
  rdivide/1 -> Out1/1

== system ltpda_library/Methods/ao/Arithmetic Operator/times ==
  In1 : Inport  OutDataType=sfix(16)  OutScaling=2^0
  times : M-S-Function  Tag=times  FunctionName=ltpdasim
  Out1 : Outport  OutDataType=sfix(16)  OutScaling=2^0
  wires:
  In1/1 -> times/1
  times/1 -> Out1/1

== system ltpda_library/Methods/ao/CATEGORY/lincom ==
  In1 : Inport  OutDataType=sfix(16)  OutScaling=2^0
  lincom : M-S-Function  Tag=lincom  FunctionName=ltpdasim
  Out1 : Outport  OutDataType=sfix(16)  OutScaling=2^0
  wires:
  In1/1 -> lincom/1
  lincom/1 -> Out1/1

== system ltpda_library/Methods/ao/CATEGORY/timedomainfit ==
  In1 : Inport  OutDataType=sfix(16)  OutScaling=2^0
  timedomainfit : M-S-Function  Tag=timedomainfit  FunctionName=ltpdasim
  Out1 : Outport  OutDataType=sfix(16)  OutScaling=2^0
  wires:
  In1/1 -> timedomainfit/1
  timedomainfit/1 -> Out1/1

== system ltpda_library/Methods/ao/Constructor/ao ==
  Ground : Ground
  ao : M-S-Function  Tag=ao  FunctionName=ltpdasim
  Out1 : Outport  OutDataType=sfix(16)  OutScaling=2^0
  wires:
  Ground/1 -> ao/1
  ao/1 -> Out1/1

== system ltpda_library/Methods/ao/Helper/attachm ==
  In1 : Inport  OutDataType=sfix(16)  OutScaling=2^0
  attachm : M-S-Function  Tag=attachm  FunctionName=ltpdasim
  Out1 : Outport  OutDataType=sfix(16)  OutScaling=2^0
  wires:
  In1/1 -> attachm/1
  attachm/1 -> Out1/1

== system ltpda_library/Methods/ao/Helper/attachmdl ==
  In1 : Inport  OutDataType=sfix(16)  OutScaling=2^0
  attachmdl : M-S-Function  Tag=attachmdl  FunctionName=ltpdasim
  Out1 : Outport  OutDataType=sfix(16)  OutScaling=2^0
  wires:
  In1/1 -> attachmdl/1
  attachmdl/1 -> Out1/1

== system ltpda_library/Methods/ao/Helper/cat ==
  In1 : Inport  OutDataType=sfix(16)  OutScaling=2^0
  cat : M-S-Function  Tag=cat  FunctionName=ltpdasim
  Out1 : Outport  OutDataType=sfix(16)  OutScaling=2^0
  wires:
  In1/1 -> cat/1
  cat/1 -> Out1/1

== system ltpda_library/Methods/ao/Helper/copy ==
  In1 : Inport  OutDataType=sfix(16)  OutScaling=2^0
  copy : M-S-Function  Tag=copy  FunctionName=ltpdasim
  Out1 : Outport  OutDataType=sfix(16)  OutScaling=2^0
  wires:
  In1/1 -> copy/1
  copy/1 -> Out1/1

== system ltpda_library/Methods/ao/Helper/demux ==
  In1 : Inport  OutDataType=sfix(16)  OutScaling=2^0
  demux : M-S-Function  Tag=demux  FunctionName=ltpdasim
  Out1 : Outport  OutDataType=sfix(16)  OutScaling=2^0
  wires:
  In1/1 -> demux/1
  demux/1 -> Out1/1

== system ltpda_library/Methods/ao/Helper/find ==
  In1 : Inport  OutDataType=sfix(16)  OutScaling=2^0
  find : M-S-Function  Tag=find  FunctionName=ltpdasim
  Out1 : Outport  OutDataType=sfix(16)  OutScaling=2^0
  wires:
  In1/1 -> find/1
  find/1 -> Out1/1

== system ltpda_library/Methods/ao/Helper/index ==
  In1 : Inport  OutDataType=sfix(16)  OutScaling=2^0
  index : M-S-Function  Tag=index  FunctionName=ltpdasim
  Out1 : Outport  OutDataType=sfix(16)  OutScaling=2^0
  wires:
  In1/1 -> index/1
  index/1 -> Out1/1

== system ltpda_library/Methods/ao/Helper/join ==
  In1 : Inport  OutDataType=sfix(16)  OutScaling=2^0
  join : M-S-Function  Tag=join  FunctionName=ltpdasim
  Out1 : Outport  OutDataType=sfix(16)  OutScaling=2^0
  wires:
  In1/1 -> join/1
  join/1 -> Out1/1

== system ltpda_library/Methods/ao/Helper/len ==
  In1 : Inport  OutDataType=sfix(16)  OutScaling=2^0
  len : M-S-Function  Tag=len  FunctionName=ltpdasim
  Out1 : Outport  OutDataType=sfix(16)  OutScaling=2^0
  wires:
  In1/1 -> len/1
  len/1 -> Out1/1

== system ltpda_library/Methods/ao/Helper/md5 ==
  In1 : Inport  OutDataType=sfix(16)  OutScaling=2^0
  md5 : M-S-Function  Tag=md5  FunctionName=ltpdasim
  Out1 : Outport  OutDataType=sfix(16)  OutScaling=2^0
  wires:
  In1/1 -> md5/1
  md5/1 -> Out1/1

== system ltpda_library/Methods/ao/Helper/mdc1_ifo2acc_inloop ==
  In1 : Inport  OutDataType=sfix(16)  OutScaling=2^0
  mdc1_ifo2acc_inloop : M-S-Function  Tag=mdc1_ifo2acc_inloop  FunctionName=ltpdasim
  Out1 : Outport  OutDataType=sfix(16)  OutScaling=2^0
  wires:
  In1/1 -> mdc1_ifo2acc_inloop/1
  mdc1_ifo2acc_inloop/1 -> Out1/1

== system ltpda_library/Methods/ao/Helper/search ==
  In1 : Inport  OutDataType=sfix(16)  OutScaling=2^0
  search : M-S-Function  Tag=search  FunctionName=ltpdasim
  Out1 : Outport  OutDataType=sfix(16)  OutScaling=2^0
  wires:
  In1/1 -> search/1
  search/1 -> Out1/1

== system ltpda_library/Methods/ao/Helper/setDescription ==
  In1 : Inport  OutDataType=sfix(16)  OutScaling=2^0
  setDescription : M-S-Function  Tag=setDescription  FunctionName=ltpdasim
  Out1 : Outport  OutDataType=sfix(16)  OutScaling=2^0
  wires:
  In1/1 -> setDescription/1
  setDescription/1 -> Out1/1

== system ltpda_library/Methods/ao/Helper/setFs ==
  In1 : Inport  OutDataType=sfix(16)  OutScaling=2^0
  setFs : M-S-Function  Tag=setFs  FunctionName=ltpdasim
  Out1 : Outport  OutDataType=sfix(16)  OutScaling=2^0
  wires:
  In1/1 -> setFs/1
  setFs/1 -> Out1/1

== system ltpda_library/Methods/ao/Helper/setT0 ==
  In1 : Inport  OutDataType=sfix(16)  OutScaling=2^0
  setT0 : M-S-Function  Tag=setT0  FunctionName=ltpdasim
  Out1 : Outport  OutDataType=sfix(16)  OutScaling=2^0
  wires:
  In1/1 -> setT0/1
  setT0/1 -> Out1/1

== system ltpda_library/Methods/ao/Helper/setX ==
  In1 : Inport  OutDataType=sfix(16)  OutScaling=2^0
  setX : M-S-Function  Tag=setX  FunctionName=ltpdasim
  Out1 : Outport  OutDataType=sfix(16)  OutScaling=2^0
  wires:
  In1/1 -> setX/1
  setX/1 -> Out1/1

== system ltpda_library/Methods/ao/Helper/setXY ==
  In1 : Inport  OutDataType=sfix(16)  OutScaling=2^0
  setXY : M-S-Function  Tag=setXY  FunctionName=ltpdasim
  Out1 : Outport  OutDataType=sfix(16)  OutScaling=2^0
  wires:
  In1/1 -> setXY/1
  setXY/1 -> Out1/1

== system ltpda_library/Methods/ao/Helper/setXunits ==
  In1 : Inport  OutDataType=sfix(16)  OutScaling=2^0
  setXunits : M-S-Function  Tag=setXunits  FunctionName=ltpdasim
  Out1 : Outport  OutDataType=sfix(16)  OutScaling=2^0
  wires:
  In1/1 -> setXunits/1
  setXunits/1 -> Out1/1

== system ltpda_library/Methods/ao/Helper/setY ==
  In1 : Inport  OutDataType=sfix(16)  OutScaling=2^0
  setY : M-S-Function  Tag=setY  FunctionName=ltpdasim
  Out1 : Outport  OutDataType=sfix(16)  OutScaling=2^0
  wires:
  In1/1 -> setY/1
  setY/1 -> Out1/1

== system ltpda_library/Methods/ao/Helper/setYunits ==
  In1 : Inport  OutDataType=sfix(16)  OutScaling=2^0
  setYunits : M-S-Function  Tag=setYunits  FunctionName=ltpdasim
  Out1 : Outport  OutDataType=sfix(16)  OutScaling=2^0
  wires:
  In1/1 -> setYunits/1
  setYunits/1 -> Out1/1

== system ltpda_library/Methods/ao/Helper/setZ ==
  In1 : Inport  OutDataType=sfix(16)  OutScaling=2^0
  setZ : M-S-Function  Tag=setZ  FunctionName=ltpdasim
  Out1 : Outport  OutDataType=sfix(16)  OutScaling=2^0
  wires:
  In1/1 -> setZ/1
  setZ/1 -> Out1/1

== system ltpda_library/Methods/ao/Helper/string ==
  In1 : Inport  OutDataType=sfix(16)  OutScaling=2^0
  string : M-S-Function  Tag=string  FunctionName=ltpdasim
  Out1 : Outport  OutDataType=sfix(16)  OutScaling=2^0
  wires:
  In1/1 -> string/1
  string/1 -> Out1/1

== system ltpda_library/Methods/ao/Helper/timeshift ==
  In1 : Inport  OutDataType=sfix(16)  OutScaling=2^0
  timeshift : M-S-Function  Tag=timeshift  FunctionName=ltpdasim
  Out1 : Outport  OutDataType=sfix(16)  OutScaling=2^0
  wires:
  In1/1 -> timeshift/1
  timeshift/1 -> Out1/1

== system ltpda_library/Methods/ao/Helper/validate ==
  In1 : Inport  OutDataType=sfix(16)  OutScaling=2^0
  validate : M-S-Function  Tag=validate  FunctionName=ltpdasim
  Out1 : Outport  OutDataType=sfix(16)  OutScaling=2^0
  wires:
  In1/1 -> validate/1
  validate/1 -> Out1/1

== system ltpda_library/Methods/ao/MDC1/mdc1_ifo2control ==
  In1 : Inport  OutDataType=sfix(16)  OutScaling=2^0
  mdc1_ifo2control : M-S-Function  Tag=mdc1_ifo2control  FunctionName=ltpdasim
  Out1 : Outport  OutDataType=sfix(16)  OutScaling=2^0
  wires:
  In1/1 -> mdc1_ifo2control/1
  mdc1_ifo2control/1 -> Out1/1

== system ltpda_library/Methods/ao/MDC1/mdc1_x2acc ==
  In1 : Inport  OutDataType=sfix(16)  OutScaling=2^0
  mdc1_x2acc : M-S-Function  Tag=mdc1_x2acc  FunctionName=ltpdasim
  Out1 : Outport  OutDataType=sfix(16)  OutScaling=2^0
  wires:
  In1/1 -> mdc1_x2acc/1
  mdc1_x2acc/1 -> Out1/1

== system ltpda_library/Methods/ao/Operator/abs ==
  In1 : Inport  OutDataType=sfix(16)  OutScaling=2^0
  abs : M-S-Function  Tag=abs  FunctionName=ltpdasim
  Out1 : Outport  OutDataType=sfix(16)  OutScaling=2^0
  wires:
  In1/1 -> abs/1
  abs/1 -> Out1/1

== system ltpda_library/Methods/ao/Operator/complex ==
  In1 : Inport  OutDataType=sfix(16)  OutScaling=2^0
  complex : M-S-Function  Tag=complex  FunctionName=ltpdasim
  Out1 : Outport  OutDataType=sfix(16)  OutScaling=2^0
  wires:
  In1/1 -> complex/1
  complex/1 -> Out1/1

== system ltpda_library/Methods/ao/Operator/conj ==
  In1 : Inport  OutDataType=sfix(16)  OutScaling=2^0
  conj : M-S-Function  Tag=conj  FunctionName=ltpdasim
  Out1 : Outport  OutDataType=sfix(16)  OutScaling=2^0
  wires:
  In1/1 -> conj/1
  conj/1 -> Out1/1

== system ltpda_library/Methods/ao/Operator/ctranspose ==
  In1 : Inport  OutDataType=sfix(16)  OutScaling=2^0
  ctranspose : M-S-Function  Tag=ctranspose  FunctionName=ltpdasim
  Out1 : Outport  OutDataType=sfix(16)  OutScaling=2^0
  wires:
  In1/1 -> ctranspose/1
  ctranspose/1 -> Out1/1

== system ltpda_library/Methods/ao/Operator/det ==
  In1 : Inport  OutDataType=sfix(16)  OutScaling=2^0
  det : M-S-Function  Tag=det  FunctionName=ltpdasim
  Out1 : Outport  OutDataType=sfix(16)  OutScaling=2^0
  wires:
  In1/1 -> det/1
  det/1 -> Out1/1

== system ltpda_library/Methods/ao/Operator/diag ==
  In1 : Inport  OutDataType=sfix(16)  OutScaling=2^0
  diag : M-S-Function  Tag=diag  FunctionName=ltpdasim
  Out1 : Outport  OutDataType=sfix(16)  OutScaling=2^0
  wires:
  In1/1 -> diag/1
  diag/1 -> Out1/1

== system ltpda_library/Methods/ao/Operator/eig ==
  In1 : Inport  OutDataType=sfix(16)  OutScaling=2^0
  eig : M-S-Function  Tag=eig  FunctionName=ltpdasim
  Out1 : Outport  OutDataType=sfix(16)  OutScaling=2^0
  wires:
  In1/1 -> eig/1
  eig/1 -> Out1/1

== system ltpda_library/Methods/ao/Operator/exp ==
  In1 : Inport  OutDataType=sfix(16)  OutScaling=2^0
  exp : M-S-Function  Tag=exp  FunctionName=ltpdasim
  Out1 : Outport  OutDataType=sfix(16)  OutScaling=2^0
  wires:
  In1/1 -> exp/1
  exp/1 -> Out1/1

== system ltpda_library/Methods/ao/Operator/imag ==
  In1 : Inport  OutDataType=sfix(16)  OutScaling=2^0
  imag : M-S-Function  Tag=imag  FunctionName=ltpdasim
  Out1 : Outport  OutDataType=sfix(16)  OutScaling=2^0
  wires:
  In1/1 -> imag/1
  imag/1 -> Out1/1

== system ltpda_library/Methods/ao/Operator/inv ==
  In1 : Inport  OutDataType=sfix(16)  OutScaling=2^0
  inv : M-S-Function  Tag=inv  FunctionName=ltpdasim
  Out1 : Outport  OutDataType=sfix(16)  OutScaling=2^0
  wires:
  In1/1 -> inv/1
  inv/1 -> Out1/1

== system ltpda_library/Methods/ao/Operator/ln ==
  In1 : Inport  OutDataType=sfix(16)  OutScaling=2^0
  ln : M-S-Function  Tag=ln  FunctionName=ltpdasim
  Out1 : Outport  OutDataType=sfix(16)  OutScaling=2^0
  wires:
  In1/1 -> ln/1
  ln/1 -> Out1/1

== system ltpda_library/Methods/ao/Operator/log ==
  In1 : Inport  OutDataType=sfix(16)  OutScaling=2^0
  log : M-S-Function  Tag=log  FunctionName=ltpdasim
  Out1 : Outport  OutDataType=sfix(16)  OutScaling=2^0
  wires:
  In1/1 -> log/1
  log/1 -> Out1/1

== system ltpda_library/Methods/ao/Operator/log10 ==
  In1 : Inport  OutDataType=sfix(16)  OutScaling=2^0
  log10 : M-S-Function  Tag=log10  FunctionName=ltpdasim
  Out1 : Outport  OutDataType=sfix(16)  OutScaling=2^0
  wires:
  In1/1 -> log10/1
  log10/1 -> Out1/1

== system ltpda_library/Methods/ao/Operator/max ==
  In1 : Inport  OutDataType=sfix(16)  OutScaling=2^0
  max : M-S-Function  Tag=max  FunctionName=ltpdasim
  Out1 : Outport  OutDataType=sfix(16)  OutScaling=2^0
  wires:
  In1/1 -> max/1
  max/1 -> Out1/1

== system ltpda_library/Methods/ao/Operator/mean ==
  In1 : Inport  OutDataType=sfix(16)  OutScaling=2^0
  mean : M-S-Function  Tag=mean  FunctionName=ltpdasim
  Out1 : Outport  OutDataType=sfix(16)  OutScaling=2^0
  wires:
  In1/1 -> mean/1
  mean/1 -> Out1/1

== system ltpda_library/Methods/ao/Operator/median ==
  In1 : Inport  OutDataType=sfix(16)  OutScaling=2^0
  median : M-S-Function  Tag=median  FunctionName=ltpdasim
  Out1 : Outport  OutDataType=sfix(16)  OutScaling=2^0
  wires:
  In1/1 -> median/1
  median/1 -> Out1/1

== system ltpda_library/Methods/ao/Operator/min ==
  In1 : Inport  OutDataType=sfix(16)  OutScaling=2^0
  min : M-S-Function  Tag=min  FunctionName=ltpdasim
  Out1 : Outport  OutDataType=sfix(16)  OutScaling=2^0
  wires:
  In1/1 -> min/1
  min/1 -> Out1/1

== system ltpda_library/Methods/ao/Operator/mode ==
  In1 : Inport  OutDataType=sfix(16)  OutScaling=2^0
  mode : M-S-Function  Tag=mode  FunctionName=ltpdasim
  Out1 : Outport  OutDataType=sfix(16)  OutScaling=2^0
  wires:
  In1/1 -> mode/1
  mode/1 -> Out1/1

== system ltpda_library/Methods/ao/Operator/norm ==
  In1 : Inport  OutDataType=sfix(16)  OutScaling=2^0
  norm : M-S-Function  Tag=norm  FunctionName=ltpdasim
  Out1 : Outport  OutDataType=sfix(16)  OutScaling=2^0
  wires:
  In1/1 -> norm/1
  norm/1 -> Out1/1

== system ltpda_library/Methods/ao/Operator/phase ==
  In1 : Inport  OutDataType=sfix(16)  OutScaling=2^0
  phase : M-S-Function  Tag=phase  FunctionName=ltpdasim
  Out1 : Outport  OutDataType=sfix(16)  OutScaling=2^0
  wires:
  In1/1 -> phase/1
  phase/1 -> Out1/1

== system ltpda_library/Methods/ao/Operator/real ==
  In1 : Inport  OutDataType=sfix(16)  OutScaling=2^0
  real : M-S-Function  Tag=real  FunctionName=ltpdasim
  Out1 : Outport  OutDataType=sfix(16)  OutScaling=2^0
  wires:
  In1/1 -> real/1
  real/1 -> Out1/1

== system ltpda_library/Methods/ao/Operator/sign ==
  In1 : Inport  OutDataType=sfix(16)  OutScaling=2^0
  sign : M-S-Function  Tag=sign  FunctionName=ltpdasim
  Out1 : Outport  OutDataType=sfix(16)  OutScaling=2^0
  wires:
  In1/1 -> sign/1
  sign/1 -> Out1/1

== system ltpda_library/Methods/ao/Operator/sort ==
  In1 : Inport  OutDataType=sfix(16)  OutScaling=2^0
  sort : M-S-Function  Tag=sort  FunctionName=ltpdasim
  Out1 : Outport  OutDataType=sfix(16)  OutScaling=2^0
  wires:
  In1/1 -> sort/1
  sort/1 -> Out1/1
